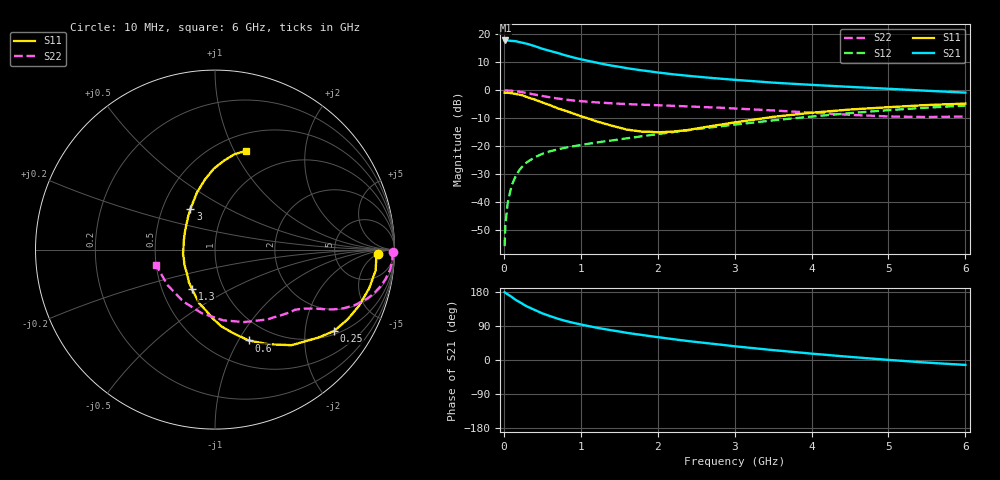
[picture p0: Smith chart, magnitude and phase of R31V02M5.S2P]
! SIEMENS Small Signal Semiconductors
! BFR181
! Si NPN RF Bipolar Junction Transistor in SOT23
! VCE = 1 V  IC = 2.5 mA
! Common Emitter S-Parameters:  May  1996
# GHz  S  MA  R  50
!  f  S11  S21  S12  S22
! GHz  MAG  ANG  MAG  ANG  MAG  ANG  MAG  ANG
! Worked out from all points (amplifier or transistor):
!   36 points, 10 MHz to 6 GHz, reference 50 ohm
!   highest |S21| = 17.9 dB at 20 MHz (marker M1)
!   |S21| within 3 dB of that: start of sweep to 502.3 MHz
!   unconditionally stable (mu >= 1): 1.366 GHz to 3.436 GHz
!   at 250 MHz: K = 0.28, MSG = 22.0 dB, |S12| = -27.1 dB
!   at 1.4 GHz: K = 1.01, MAG = 12.8 dB, |S12| = -18.0 dB
!   at 6 GHz: K = 0.89, MSG = 2.3 dB, |S12| = -5.5 dB
!   S11 on the Smith chart (normalised r, x): 10 MHz: 19, -5; 250 MHz: 1.11, -2.84; 600 MHz: 0.77, -1.10; 1.3 GHz: 0.71, -0.33; 3 GHz: 0.69, +0.34; 6 GHz: 0.68, +1.12
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0.01  0.9064 -1.6  7.753 178.9  0.0016 88.6  0.9945 -0.7
0.02  0.8997 -2.8  7.818 177.2  0.0038 87.2  0.9893 -1.4
0.05  0.9026 -7.3  7.813 173.3  0.0096 86.5  0.9903 -3.5
0.1  0.8857 -14.1  7.666 166.8  0.0193 82.0  0.9813 -6.7
0.15  0.8609 -21.4  7.597 159.2  0.0281 76.6  0.9624 -10.1
0.25  0.8034 -34.4  7.066 147.3  0.0444 70.5  0.9176 -15.5
0.3  0.7548 -40.6  6.818 141.4  0.0512 68.4  0.8903 -17.9
0.4  0.6824 -51.3  6.201 132.2  0.0627 63.3  0.8374 -21.7
0.5  0.6046 -60.7  5.546 123.1  0.0724 59.9  0.7896 -24.4
0.6  0.5398 -69.7  5.08 115.8  0.0805 57.3  0.7476 -26.4
0.7  0.4753 -77.9  4.655 109.1  0.087 55.6  0.7111 -28.0
0.8  0.4287 -85.3  4.234 103.2  0.0933 54.5  0.6809 -29.1
0.9  0.3846 -91.8  3.884 98.2  0.0987 53.9  0.6564 -30.1
1.1  0.311 -106.6  3.36 89.6  0.1098 53.5  0.6215 -31.9
1.3  0.2544 -120.3  2.936 81.9  0.1208 53.5  0.5951 -33.6
1.7  0.1888 -154.9  2.374 68.7  0.1434 55.0  0.5568 -37.1
2.2  0.1812 163.3  1.934 55.0  0.1775 55.3  0.5254 -43.4
3  0.2648 121.1  1.539 36.2  0.2419 53.2  0.471 -56.5
3.5  0.3333 107.6  1.37 26.1  0.2883 50.0  0.4347 -68.3
4.5  0.4514 90.8  1.149 8.2  0.3888 40.6  0.3628 -101.4
5.5  0.543 78.4  0.979 -6.9  0.4877 28.0  0.3306 -143.6
6  0.5771 72.4  0.908 -13.0  0.5307 20.8  0.3384 -165.3
